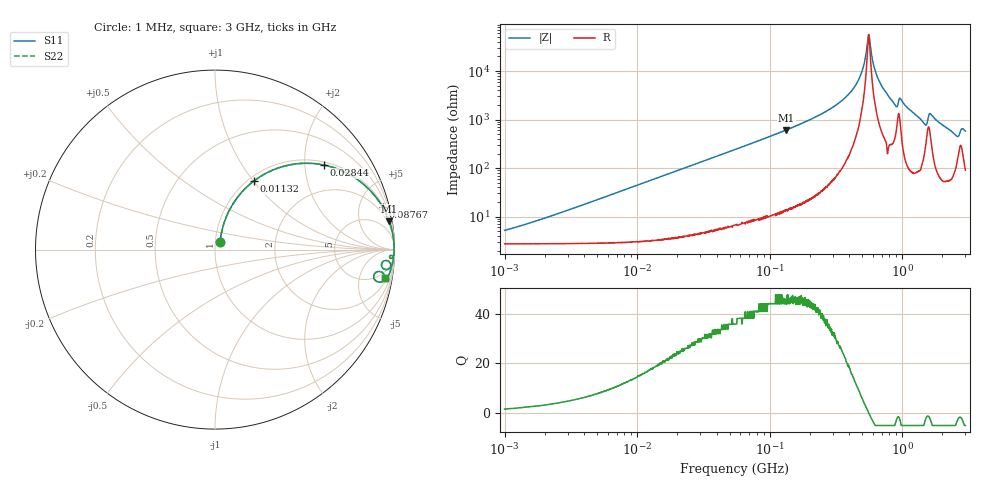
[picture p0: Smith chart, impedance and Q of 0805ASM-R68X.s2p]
!s-Parameter Generated by FASTRON Sdn. Bhd.
!FASTRON P/N : 0805ASM-R68X
!Keysight Technologies: E4991B_MY54100416_A.01.15
!Date: Fri Jun 19 14:53:14 2026
!Version  :Rev00  Fri Jun 19 14:53:14 2026
!Data & Calibration Information:
!Freq  S11  S21  S12  S22
!PortZ  Port1:50+j0  Port2:50+j0
!When reading reference impedance value at option line is always used.
! Remarks : This data is being provided solely for informational purposes.
# Hz S dB R 50
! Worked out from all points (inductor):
!   1601 points, 1 MHz to 3 GHz, reference 50 ohm
!   read as one part in series: L = 707 nH near 1.869 MHz
!   highest Q = 45.8 at 133.5 MHz (marker M1), where L = 731 nH
!   self-resonance near 558.4 MHz
!   S11 on the Smith chart (normalised r, x): 1 MHz: 1.05, +0.09; 11.32 MHz: 1.06, +1.00; 28.44 MHz: 1.09, +2.51; 87.67 MHz: 1.18, +7.80; 3 GHz: 3, -11
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1000000  -25.90 55.8  -0.24 -2.5  -0.24 -2.5  -25.90 55.8
3804036  -15.70 71.3  -0.35 -9.3  -0.35 -9.3  -15.70 71.3
1.132407e7  -7.17 60.5  -1.19 -25.9  -1.19 -25.9  -7.17 60.5
1.447069e7  -5.56 55.3  -1.69 -31.8  -1.69 -31.8  -5.56 55.3
2.843618e7  -2.28 37.8  -4.25 -50.2  -4.25 -50.2  -2.28 37.8
5.504702e7  -0.76 22.1  -8.47 -66.3  -8.47 -66.3  -0.76 22.1
8.766808e7  -0.33 14.3  -12.20 -74.4  -12.20 -74.4  -0.33 14.3
1.334721e8  -0.14 9.2  -15.90 -79.5  -15.90 -79.5  -0.14 9.2
2.083556e8  -0.06 5.5  -20.40 -83.2  -20.40 -83.2  -0.06 5.5
3.204059e8  -0.02 2.8  -26.20 -85.2  -26.20 -85.2  -0.02 2.8
4.240331e8  -0.02 1.4  -32.50 -84.8  -32.50 -84.8  -0.02 1.4
4.951867e8  -0.01 0.6  -39.60 -80.4  -39.60 -80.4  -0.01 0.6
5.583748e8  -0.02 0.0  -55.10 -6.4  -55.10 -6.4  -0.02 0.0
5.725215e8  -0.02 -0.1  -51.60 47.6  -51.60 47.6  -0.02 -0.1
6.423554e8  -0.02 -0.7  -38.30 79.9  -38.30 79.9  -0.02 -0.7
7.925923e8  -0.03 -1.9  -29.40 82.6  -29.40 82.6  -0.03 -1.9
8.937307e8  -0.13 -2.9  -25.80 72.2  -25.80 72.2  -0.13 -2.9
9.828732e8  -0.07 -2.2  -28.30 76.5  -28.30 76.5  -0.07 -2.2
1.474099e9  -0.32 -6.6  -18.50 69.1  -18.50 69.1  -0.32 -6.6
1.645649e9  -0.22 -4.1  -22.50 68.6  -22.50 68.6  -0.22 -4.1
2.530652e9  -0.52 -11.1  -14.10 67.3  -14.10 67.3  -0.52 -11.1
3e9  -0.35 -9.5  -15.60 71.5  -15.60 71.5  -0.35 -9.5
